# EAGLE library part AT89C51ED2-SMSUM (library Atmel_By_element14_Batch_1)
8-bit Flash Microcontroller
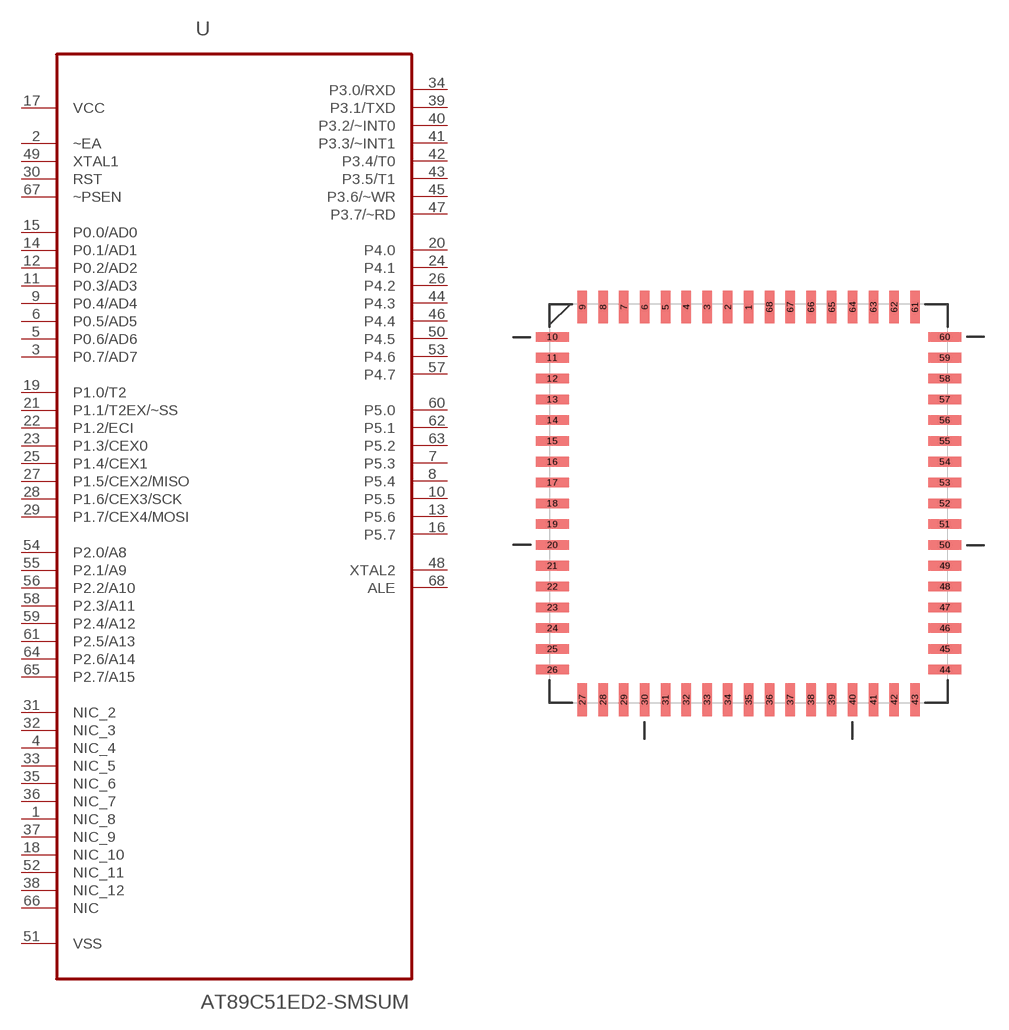
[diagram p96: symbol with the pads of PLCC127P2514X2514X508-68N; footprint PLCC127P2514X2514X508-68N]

Designator prefix U

## AT89C51ED2-SMSUM (DESCRIPTION: 8-bit Flash Microcontroller; MPN: AT89C51ED2-SMSUM; OC_FARNELL: 1095727; OC_NEWARK: 96K6568; PACKAGE: PLCC-68; SUPPLIER: Atmel)  [PLCC127P2514X2514X508-68N]
1  NIC_8  nc
2  ~EA  in
3  P0.7/AD7
4  NIC_4  nc
5  P0.6/AD6
6  P0.5/AD5
7  P5.3
8  P5.4
9  P0.4/AD4
10  P5.5
11  P0.3/AD3
12  P0.2/AD2
13  P5.6
14  P0.1/AD1
15  P0.0/AD0
16  P5.7
17  VCC  pwr
18  NIC_10  nc
19  P1.0/T2
20  P4.0
21  P1.1/T2EX/~SS
22  P1.2/ECI
23  P1.3/CEX0
24  P4.1
25  P1.4/CEX1
26  P4.2
27  P1.5/CEX2/MISO
28  P1.6/CEX3/SCK
29  P1.7/CEX4/MOSI
30  RST  in
31  NIC_2  nc
32  NIC_3  nc
33  NIC_5  nc
34  P3.0/RXD
35  NIC_6  nc
36  NIC_7  nc
37  NIC_9  nc
38  NIC_12  nc
39  P3.1/TXD
40  P3.2/~INT0
41  P3.3/~INT1
42  P3.4/T0
43  P3.5/T1
44  P4.3
45  P3.6/~WR
46  P4.4
47  P3.7/~RD
48  XTAL2  out
49  XTAL1  in
50  P4.5
51  VSS  pwr
52  NIC_11  nc
53  P4.6
54  P2.0/A8
55  P2.1/A9
56  P2.2/A10
57  P4.7
58  P2.3/A11
59  P2.4/A12
60  P5.0
61  P2.5/A13
62  P5.1
63  P5.2
64  P2.6/A14
65  P2.7/A15
66  NIC  nc
67  ~PSEN  in
68  ALE  out

## Footprint PLCC127P2514X2514X508-68N (pad centres in mm)
smd 0.584 x 2.007: 1 0,11.989; 2 -1.27,11.989; 3 -2.54,11.989; 4 -3.81,11.989; 5 -5.08,11.989; 6 -6.35,11.989; 7 -7.62,11.989; 8 -8.89,11.989; 9 -10.16,11.989; 27 -10.16,-11.989; 28 -8.89,-11.989; 29 -7.62,-11.989; 30 -6.35,-11.989; 31 -5.08,-11.989; 32 -3.81,-11.989; 33 -2.54,-11.989; 34 -1.27,-11.989; 35 0,-11.989; 36 1.27,-11.989; 37 2.54,-11.989; 38 3.81,-11.989; 39 5.08,-11.989; 40 6.35,-11.989; 41 7.62,-11.989; 42 8.89,-11.989; 43 10.16,-11.989; 61 10.16,11.989; 62 8.89,11.989; 63 7.62,11.989; 64 6.35,11.989; 65 5.08,11.989; 66 3.81,11.989; 67 2.54,11.989; 68 1.27,11.989
smd 2.007 x 0.584: 10 -11.989,10.16; 11 -11.989,8.89; 12 -11.989,7.62; 13 -11.989,6.35; 14 -11.989,5.08; 15 -11.989,3.81; 16 -11.989,2.54; 17 -11.989,1.27; 18 -11.989,0; 19 -11.989,-1.27; 20 -11.989,-2.54; 21 -11.989,-3.81; 22 -11.989,-5.08; 23 -11.989,-6.35; 24 -11.989,-7.62; 25 -11.989,-8.89; 26 -11.989,-10.16; 44 11.989,-10.16; 45 11.989,-8.89; 46 11.989,-7.62; 47 11.989,-6.35; 48 11.989,-5.08; 49 11.989,-3.81; 50 11.989,-2.54; 51 11.989,-1.27; 52 11.989,0; 53 11.989,1.27; 54 11.989,2.54; 55 11.989,3.81; 56 11.989,5.08; 57 11.989,6.35; 58 11.989,7.62; 59 11.989,8.89; 60 11.989,10.16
